(* This function block represents one IEC 60870-5-101 slave->master connection channel *)
FUNCTION_BLOCK FB_IEC870_5_101S
VAR_IN_OUT
	hSerial		: T_HSERIALCTRL;(* Serial connection control handle *)
	stProcData	: ST_IEC870_5_101SProcData;(* Process data send to or received from IEC 60870-5-101 master device *)
	fbLog		: FB_IEC870_DebugLogFifo;(* Simple log buffer. We store/log here all our received slave data and other messages *)
END_VAR
VAR_INPUT
	protPara	: ST_IEC870_5_101ProtocolParams := ( eType := eIEC870_101_SLAVE );(* Serial link transport protocol parameters *)
	sysPara		: ST_IEC870_5_101SSysPara;(* System parameter *)
	bEnable		: BOOL := TRUE; (* Enables/disables communication channel *)
END_VAR
VAR
	fbProtocol	: FB_IEC870_5_101TProtocol;(* IEC60870-5-101 transport *)
	fbServices	: FB_IEC870_5_101SServices;(* IEC60870-5-101 slave services *)
	fbClock		: FB_LocalSystemTime;(* Internal clock: Local windows system time *)
	buffer		: ST_IEC870_5_101TBuffer;(* TX/RX data buffer *)
	nState		: BYTE;
	bReset 		: BOOL;(* Rising edge at this input resets service execution *)
END_VAR

fbClock( bEnable := TRUE, dwCycle := 1 );(* Get local Windows System Time *)
IF NOT fbClock.bValid THEN
	RETURN;
END_IF


CASE nState OF
	0:	(* Init step *)
		IF bEnable THEN
			(* Enable/disable application layer messages *)
			fbLog( sPrefix :=CONCAT( 'IEC 60870-5-101S, linkAddr:', CONCAT( DWORD_TO_STRING( protPara.linkAddr ), CONCAT( ', CAA:', DWORD_TO_STRING( sysPara.asduAddr ) ) ) ) );

			(* Initialize the max. asdu size, frame format params and buffer debug mode *)
			buffer.eDbg 	:= sysPara.eDbgAsdu;(* Enable/disable debug output of asdu data *)
			buffer.asduSize	:= F_iecApdu101ToAsduLen( fbProtocol.protPara.FRAMELength, fbProtocol.protPara.eLinkAddrSize );
			buffer.asduFmt	:= sysPara.asduFmt;(* Set the frame format parameters (octet sizes) *)
			bReset 			:= TRUE;(* Set flag => reset service execution *)

			(* Reset protocol function block and restart data transfer *)
			fbProtocol.INIT( hSerial := hSerial, buffer	:= buffer, protPara := protPara, bOutDbg := sysPara.bDbgLink );
			nState := 1;
		END_IF

	1: (* Establish connection and exchange data *)
		IF bEnable THEN
			fbProtocol( hSerial := hSerial, buffer := buffer );
			IF NOT fbProtocol.bError THEN
				IF fbProtocol.eState = eSERIALLINK_ESTABLISHED THEN

					(* Link established => exchange data *)
					fbServices( buffer := buffer, sysPara := sysPara, bReset := bReset, stProcData := stProcData, fbClock := fbClock, fbLog := fbLog );

				END_IF
			ELSE (* Error => reset connection *)
				fbLog.A_LogError( sPut := CONCAT( '::Transport interface error: 0x', DWORD_TO_HEXSTR( fbProtocol.nErrID, 8, TRUE ) ) );
				nState := 0;
			END_IF
		ELSE (* Stop communication *)
			nState := 0;
		END_IF
END_CASE

END_FUNCTION_BLOCK
